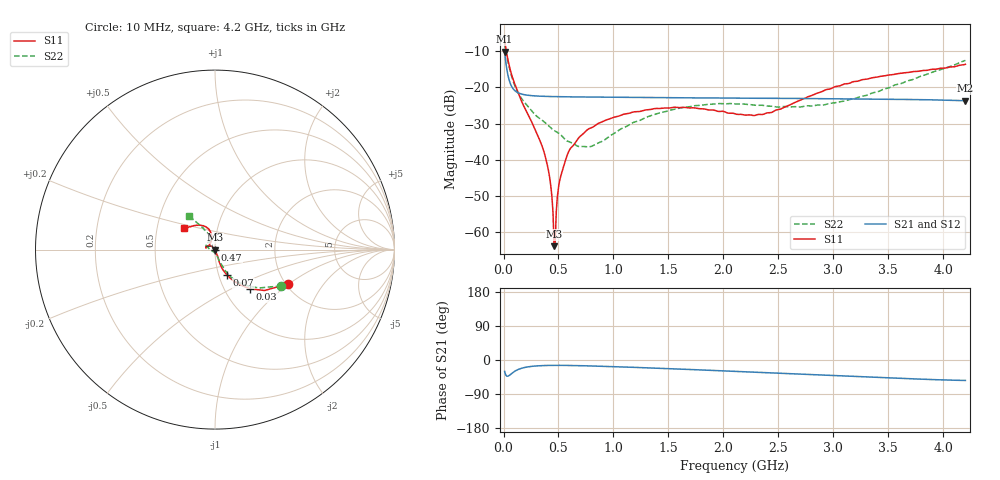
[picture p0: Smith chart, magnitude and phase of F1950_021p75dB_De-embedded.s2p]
! Integrated Device Technology
! Corporate Headquarters
! 6024 Silver Creek Valley Road
! San Jose, CA 95138  USA
! Phone:  1-408-284-8200
! Toll Free:  1-800-223-1366
! Webpage:  http://www.idt.com/
! Timing and RF Division
! 515 Groton Road, Suite 102
! Westford, MA 01886-6024
! Device:  F1950
! Description: 7-bit 0.25 dB Digital Step Attenuator
! Frequency:  150.0 -  4000.00 MHz
! Package:  4x4 mm Thin QFN Plastic Package: 24 pin
! Ports:  2 RF, 12 DC
!  Pin  1  = D0
!  Pin  2  = VDD
!  Pin  3  = Vmode
!  Pin  4  = GND
!  Pin  5  = RF1  =  Port 1
!  Pin  6  = GND
!  Pin  7  = GND
!  Pin  8  = GND
!  Pin  9  = GND
!  Pin 10  = GND
!  Pin 11  = GND
!  Pin 12  = GND
!  Pin 13  = GND
!  Pin 14  = RF2  =  Port 2
!  Pin 15  = GND
!  Pin 16  = LE
!  Pin 17  = CLK
!  Pin 18  = DATE
!  Pin 19  = D6
!  Pin 20  = D5
!  Pin 21  = D4
!  Pin 22  = D3
!  Pin 23  = D2
!  Pin 24  = D1
! State:  87
! Atten State:  21.75 dB
! Voltage:  +5.00 Volts
! Current:  Not Measured mA
! Data:  The device was measured on a the F195X evaluation board which has
!  individual transmission lines to the RF pins.  Data was collected
!  using a calibrated network analyzer.  The evaluation board was
!  de-embedded using a TRL calibration technique.
!  The reference plane is the edge of the package pin.
! Misc:  Board 2019
!  Action Tracker AT0250
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# GHz S dB R 50
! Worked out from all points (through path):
!   420 points, 10 MHz to 4.2 GHz, reference 50 ohm
!   highest |S21| = -10.12 dB at 10 MHz (marker M1); lowest = -23.7 dB at 4.2 GHz (marker M2)
!   group delay of S21, straight-line fit = 27.1 ps
!   lowest |S11| = -64.0 dB at 460 MHz (marker M3), VSWR 1.00, Z = 50 - j0.0633 ohm
!   |S11| at or under -10 dB: 26.15 MHz to end of sweep
!   |S22| runs from -36.5 to -7.5 dB; largest |S21 - S12| = 0.00014
!   S11 on the Smith chart (normalised r, x): 10 MHz: 2.04, -0.98; 30 MHz: 1.31, -0.63; 70 MHz: 1.10, -0.32; 470 MHz: 1.00, +0.00; 4.2 GHz: 0.69, +0.17
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0.01  -6.99 -25.4  -10.12 -30.0  -10.12 -30.0  -7.51 -28.7
0.03  -10.68 -48.4  -14.92 -42.7  -14.92 -42.7  -11.46 -48.8
0.07  -16.10 -64.7  -19.50 -36.6  -19.50 -36.6  -16.51 -62.6
0.16  -23.52 -70.7  -21.80 -22.2  -21.80 -22.2  -22.87 -69.0
0.37  -38.04 -63.2  -22.47 -14.6  -22.47 -14.6  -29.55 -74.1
0.42  -45.01 -66.3  -22.51 -14.2  -22.52 -14.3  -30.88 -75.4
0.45  -54.55 -70.2  -22.54 -14.1  -22.54 -14.1  -31.70 -78.7
0.46  -63.97 -88.7  -22.54 -14.1  -22.54 -14.1  -31.92 -80.1
0.47  -62.99 136.4  -22.55 -14.1  -22.55 -14.1  -32.10 -81.4
0.48  -54.36 129.1  -22.55 -14.1  -22.55 -14.1  -32.28 -82.4
0.5  -47.73 128.1  -22.57 -14.1  -22.57 -14.1  -32.64 -83.8
0.51  -45.91 129.7  -22.57 -14.1  -22.57 -14.1  -32.84 -84.3
0.55  -41.56 129.4  -22.59 -14.2  -22.59 -14.2  -34.10 -87.4
0.6  -37.31 131.5  -22.61 -14.4  -22.61 -14.4  -35.09 -98.0
0.71  -33.22 135.0  -22.65 -15.0  -22.65 -15.0  -36.37 -119.8
0.99  -28.43 145.9  -22.74 -17.5  -22.74 -17.5  -33.03 -173.9
1.41  -25.84 162.3  -22.84 -21.9  -22.84 -21.9  -27.13 162.6
2.11  -27.36 156.9  -22.97 -30.2  -22.97 -30.2  -24.58 143.8
2.43  -26.98 124.3  -23.02 -34.0  -23.02 -34.0  -25.18 133.1
2.81  -22.15 103.8  -23.09 -38.8  -23.08 -38.9  -25.13 117.3
3.51  -16.53 116.6  -23.26 -47.4  -23.26 -47.5  -20.05 114.4
4.2  -13.60 145.5  -23.68 -54.0  -23.67 -54.1  -12.52 127.8
